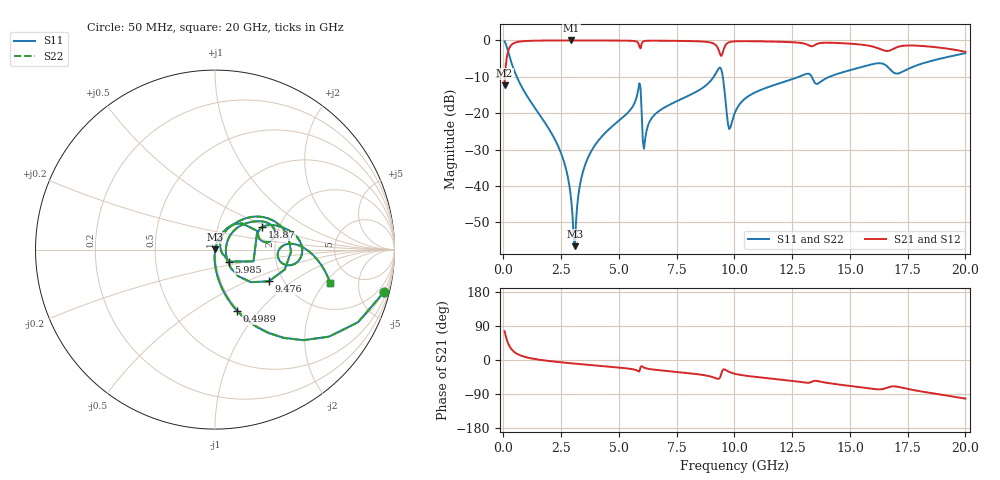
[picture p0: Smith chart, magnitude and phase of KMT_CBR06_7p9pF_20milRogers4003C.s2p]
! Data measured by Modelithics Inc. support@modelithics.com 813-866-6335
! KEMET CBR0603 7.9pF, Pad Width= 0.851mm, Pad Length= 0.64mm, Pad Gap= 0.62mm, 20mil Rogers 4003C substrate Data, January 2022
# hz S ma R 50
! 2 Port Network Data from SP1.SP block
! freq  magS11  angS11  magS21  angS21  magS12  angS12  magS22  angS22
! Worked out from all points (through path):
!   401 points, 50 MHz to 20 GHz, reference 50 ohm
!   highest |S21| = -0.01 dB at 2.943 GHz (marker M1); lowest = -12.3 dB at 50 MHz (marker M2)
!   group delay of S21, straight-line fit = 14.8 ps
!   lowest |S11| = -56.5 dB at 3.092 GHz (marker M3), VSWR 1.00, Z = 50.1 + j0.0594 ohm
!   |S11| at or under -10 dB: 579 MHz to 9.104 GHz (8.525 GHz wide, 176 % of centre); 9.495 GHz to 12.78 GHz (3.288 GHz wide, 29.5 % of centre); 13.35 GHz to 14.11 GHz (765.2 MHz wide, 5.57 % of centre)
!   |S22| runs from -56.5 to -0.3 dB; largest |S21 - S12| = 0
!   S11 on the Smith chart (normalised r, x): 50 MHz: 0.98, -7.91; 498.9 MHz: 0.98, -0.77; 5.985 GHz: 1.16, -0.16; 9.476 GHz: 1.69, -0.68; 13.87 GHz: 1.63, +0.44; 20 GHz: 3.40, -2.28
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5e7  0.97 -14.2  0.2427 75.8  0.2427 75.8  0.97 -14.2
2.495e8  0.6224 -52.2  0.7819 37.7  0.7819 37.7  0.6224 -52.2
4.98875e8  0.3635 -70.1  0.9308 19.8  0.9308 19.8  0.3635 -70.1
2.394125e9  0.0337 -93.6  0.9982 -5.5  0.9982 -5.5  0.0337 -93.6
2.74325e9  0.01541 -93.2  0.9986 -7.6  0.9986 -7.6  0.01541 -93.2
2.94275e9  0.006037 -87.1  0.9987 -8.8  0.9987 -8.8  0.006037 -87.1
3.092375e9  0.00149 23.4  0.9986 -9.6  0.9986 -9.6  0.00149 23.4
3.391625e9  0.01362 73.2  0.9985 -11.3  0.9985 -11.3  0.01362 73.2
3.94025e9  0.03547 73.4  0.9978 -14.2  0.9978 -14.2  0.03547 73.4
5.8355e9  0.2098 44.4  0.9215 -29.7  0.9215 -29.7  0.2098 44.4
5.985125e9  0.1018 -40.9  0.9065 -16.0  0.9065 -16.0  0.1018 -40.9
6.13475e9  0.04409 49.4  0.9844 -21.3  0.9844 -21.3  0.04409 49.4
6.73325e9  0.1071 61.4  0.9908 -26.9  0.9908 -26.9  0.1071 61.4
9.077375e9  0.3071 36.8  0.9115 -45.6  0.9115 -45.6  0.3071 36.8
9.476375e9  0.3479 -30.5  0.6519 -28.3  0.6519 -28.3  0.3479 -30.5
9.775625e9  0.0606 -5.2  0.945 -31.5  0.945 -31.5  0.0606 -5.2
1.0025e10  0.1022 40.7  0.9719 -36.5  0.9719 -36.5  0.1022 40.7
1.097262e10  0.1982 42.9  0.9725 -45.0  0.9725 -45.0  0.1982 42.9
1.336662e10  0.3079 8.3  0.8308 -57.0  0.8308 -57.0  0.3079 8.3
1.386538e10  0.2885 25.4  0.9288 -58.9  0.9288 -58.9  0.2885 25.4
1.670825e10  0.4108 -12.2  0.7234 -71.2  0.7234 -71.2  0.4108 -12.2
2e10  0.6677 -16.1  0.6958 -101.9  0.6958 -101.9  0.6677 -16.1
